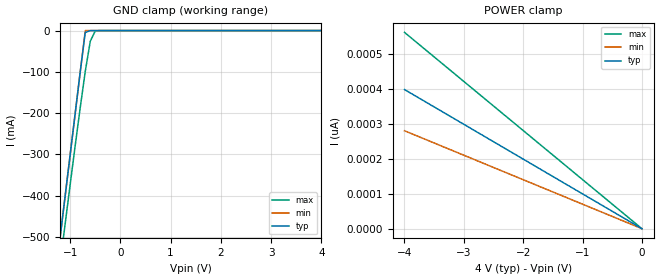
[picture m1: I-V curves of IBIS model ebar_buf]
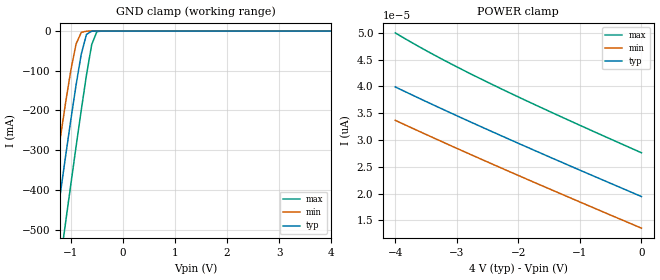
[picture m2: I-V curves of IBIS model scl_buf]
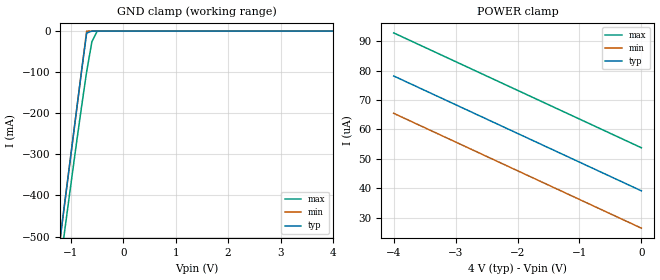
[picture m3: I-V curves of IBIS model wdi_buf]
| IBIS file m41t94.ibs created by s2ibis2 version 1.1
| North Carolina State University Electronics Research Laboratory  1995
[IBIS ver]   2.1
[File name]   m41t94.ibs
[File Rev]   0
[Date]   Apr 5, 2004
[Source]   ST models
[Copyright]   ST Microelectronics Inc.
|   Component m41t94 [Package]
[Component]   m41t94[Package]
[Manufacturer]   ST Microelectronics
[Package]
| variable   typ   min   max
R_pkg   10.0000m   10.0000m   10.0000m
L_pkg   3.0000nH   2.0000nH   4.0000nH
C_pkg   0.5000pF   0.4000pF   0.6000pF
[Pin]  signal_name   model_name   R_pin   L_pin   C_pin
vcc1   vcc1   POWER
vcc3   vcc3   POWER
vss3   vss3   GND
| dout dout   dummy
| eod  eod   dummy
| fto  fto   dummy
| sqwo sqwo   dummy
| in   dummy   dummy
1   xl   NC
2   xo   NC
3   rst#   rst_buf
4   wdi   wdi_buf
5   rstin1#   rstin_buf
6   rstin2#   rstin_buf
8   vss   GND
9   sdo   sdo_buf
10   scl   scl_buf
11   swq   sqw_buf
12   sdi   sdi_buf
13   ths   NC
14   irq#   irq_buf
15   e#   ebar_buf
16   vcc   POWER
| Models and submodels in the file (9): ebar_buf (Input), scl_buf (Input), sdi_buf (Input), wdi_buf (Input), rstin_buf (Input), rst_buf (Open_drain), sqw_buf (Output), irq_buf (Open_drain), sdo_buf (Output)
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|   Model ebar_buf
[Model]   ebar_buf
Model_type   Input
Vinl =   0.3000V
Vinh =   0.7000V
C_comp   3.2900pF   3.2200pF   4.6400pF
[Temperature Range]   27.0000   85.0000   -40.0000
[Voltage Range]   4.0000V   2.7000V   5.5000V
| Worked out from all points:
|   GND clamp passes 1 mA (typ) near -0.62 V on its own axis
[GND_clamp]
| voltage   I(typ)   I(min)   I(max)
-4V       -3.3A      -3.3A      -3.328A
-1.2V     -500mA     -500mA     -563.9mA
-1.1V     -400mA     -400mA     -467.7mA
-900mV    -200mA     -200mA     -278.2mA
-800mV    -100mA     -100mA     -186.3mA
-700mV    -4.751mA   -78.61uA   -98.9mA
-600mV    -123.9uA   -4.74uA    -25.84mA
-500mV    -3.322uA   -522.7nA   -628.6uA
4V        6.665nA    8.399nA    9.394nA
[POWER_clamp]
| voltage   I(typ)   I(min)   I(max)
-4V       398.6pA    280.5pA    562.3pA
-3.7V     368.7pA    259.5pA    520.2pA
-2.5V     249.1pA    175.3pA    351.4pA
0V        0A         0A         0A
|   Model scl_buf
[Model]   scl_buf
Model_type   Input
Vinl =   0.3000V
Vinh =   0.7000V
C_comp   3.2900pF   3.2200pF   4.6400pF
[Temperature Range]   27.0000   85.0000   -40.0000
[Voltage Range]   4.0000V   2.7000V   5.5000V
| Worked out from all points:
|   GND clamp passes 1 mA (typ) near -0.61 V on its own axis
[GND_clamp]
| voltage   I(typ)   I(min)   I(max)
-4V       -3.155A    -2.993A    -3.342A
-1.5V     -693.6mA   -545.2mA   -869.1mA
-1.4V     -597.5mA   -451.1mA   -771.5mA
-1.3V     -502mA     -358.2mA   -674.2mA
-1.2V     -407.4mA   -267.3mA   -577.3mA
-1.1V     -314.1mA   -179.5mA   -481mA
-900mV    -135.8mA   -32.42mA   -291.1mA
-800mV    -57.89mA   -3.301mA   -198.7mA
-700mV    -8.285mA   -156.8uA   -110.5mA
-600mV    -246.7uA   -9.477uA   -34.15mA
-500mV    -6.634uA   -1.045uA   -1.221mA
4V        19.44pA    19.9pA     20.03pA
[POWER_clamp]
| voltage   I(typ)   I(min)   I(max)
-4V       39.9pA     33.66pA    49.98pA
-3.7V     38.25pA    32.07pA    47.96pA
-3.3V     36.1pA     29.98pA    45.44pA
-2.5V     31.93pA    25.89pA    40.77pA
-1.4V     26.36pA    20.39pA    34.83pA
0V        19.44pA    13.54pA    27.61pA
|   Model wdi_buf
[Model]   wdi_buf
Model_type   Input
Vinl =   0.3000V
Vinh =   0.7000V
C_comp   3.0100pF   2.9400pF   3.0100pF
[Temperature Range]   27.0000   85.0000   -40.0000
[Voltage Range]   4.0000V   2.7000V   5.5000V
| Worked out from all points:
|   GND clamp passes 1 mA (typ) near -0.62 V on its own axis
[GND_clamp]
| voltage   I(typ)   I(min)   I(max)
-4V       -3.3A      -3.3A      -3.328A
-1.2V     -500mA     -500mA     -563.9mA
-1.1V     -400mA     -400mA     -467.7mA
-900mV    -200mA     -200mA     -278.2mA
-800mV    -100mA     -100mA     -186.3mA
-700mV    -4.757mA   -85.44uA   -98.9mA
-600mV    -129.8uA   -10.61uA   -25.84mA
-500mV    -8.21uA    -5.411uA   -633.3uA
4V        39.12uA    39.12uA    39.12uA
[POWER_clamp]
| voltage   I(typ)   I(min)   I(max)
-4V       78.22uA    65.51uA    92.89uA
-3.1V     69.42uA    56.71uA    84.09uA
-2.7V     65.51uA    52.8uA     80.18uA
0V        39.11uA    26.4uA     53.78uA
